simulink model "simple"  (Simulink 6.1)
settings: Solver=ode45  StartTime=0.0  StopTime=25.0  RelTol=1e-3
undefined symbols (not defined in the file or in its folder): Bit, Location, Lower, netlist, Width
libraries: xbsIndex_r3 x16, adlibrary2 x1

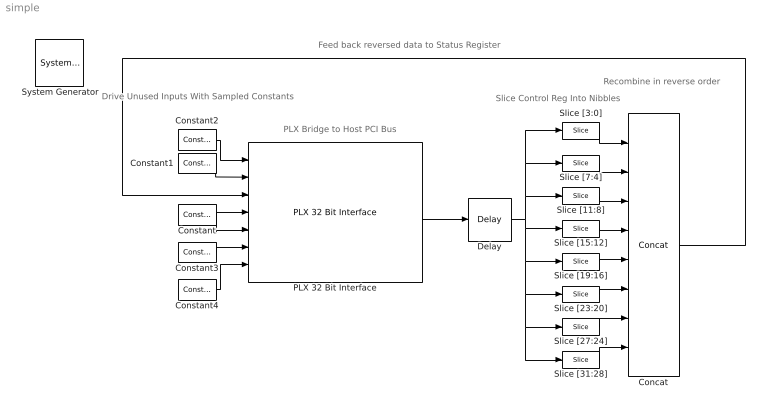
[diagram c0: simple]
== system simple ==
  note: Drive Unused Inputs With Sampled Constants
  note: PLX Bridge to Host PCI Bus
  note: Slice Control Reg Into Nibbles
  note: Recombine in reverse order
  note: Feed back reversed data to Status Register
  " System Generator" : xbsIndex_r3/ System Generator  Tag=genX  xilinxfamily=Virtex4  part=xc4vsx55  speed=-10  package=ff1148  synthesis_tool=XST  directory=./netlist  testbench=off  simulink_period=1  sysclk_period=10  incr_netlist=off  trim_vbits=Everywhere in SubSystem  dbl_ovrd=According to Block Masks  core_generation=According to Block Masks  run_coregen=off  deprecated_control=off  eval_field=0
  Concat : xbsIndex_r3/Concat  num_inputs=8  explicit_period=off  period=1  dbl_ovrd=off
  Constant : xbsIndex_r3/Constant  const=0  equ=P=C  arith_type=Boolean  n_bits=1  bin_pt=0  opselect=C  inp2=PCIN>>17  opr=+  inp1=P  carry=CIN  iostate=0  explicit_period=on  period=1  dbl_ovrd=off
  Constant1 : xbsIndex_r3/Constant  const=1  equ=P=C  arith_type=Boolean  n_bits=1  bin_pt=0  opselect=C  inp2=PCIN>>17  opr=+  inp1=P  carry=CIN  iostate=0  explicit_period=on  period=1  dbl_ovrd=off
  Constant2 : xbsIndex_r3/Constant  const=0  equ=P=C  arith_type=Unsigned  n_bits=32  bin_pt=0  opselect=C  inp2=PCIN>>17  opr=+  inp1=P  carry=CIN  iostate=0  explicit_period=on  period=1  dbl_ovrd=off
  Constant3 : xbsIndex_r3/Constant  const=0  equ=P=C  arith_type=Unsigned  n_bits=32  bin_pt=0  opselect=C  inp2=PCIN>>17  opr=+  inp1=P  carry=CIN  iostate=0  explicit_period=on  period=1  dbl_ovrd=off
  Constant4 : xbsIndex_r3/Constant  const=0  equ=P=C  arith_type=Unsigned  n_bits=34  bin_pt=0  opselect=C  inp2=PCIN>>17  opr=+  inp1=P  carry=CIN  iostate=0  explicit_period=on  period=1  dbl_ovrd=off
  Delay : xbsIndex_r3/Delay  latency=1  reg_retiming=off  explicit_period=on  period=1  en=off  accept_only_valid=off  init_zero=on  dbl_ovrd=off  show_param=off
  PLX 32 Bit Interface : adlibrary2/ADM-XRC-II/PLX 32 Bit Interface  program='slave_write 0x40000 0xabcd1234;slave_read 0x40040'  clock_ratio=1.5
  Slice [11:8] : xbsIndex_r3/Slice  mode=Lower Bit Location + Width  nbits=4  bit1=0  base1=MSB of Input  bit0=8  base0=LSB of Input  boolean_output=off  explicit_period=off  period=1  dbl_ovrd=off
  Slice [15:12] : xbsIndex_r3/Slice  mode=Lower Bit Location + Width  nbits=4  bit1=0  base1=MSB of Input  bit0=12  base0=LSB of Input  boolean_output=off  explicit_period=off  period=1  dbl_ovrd=off
  Slice [19:16] : xbsIndex_r3/Slice  mode=Lower Bit Location + Width  nbits=4  bit1=0  base1=MSB of Input  bit0=16  base0=LSB of Input  boolean_output=off  explicit_period=off  period=1  dbl_ovrd=off
  Slice [23:20] : xbsIndex_r3/Slice  mode=Lower Bit Location + Width  nbits=4  bit1=0  base1=MSB of Input  bit0=20  base0=LSB of Input  boolean_output=off  explicit_period=off  period=1  dbl_ovrd=off
  Slice [27:24] : xbsIndex_r3/Slice  mode=Lower Bit Location + Width  nbits=4  bit1=0  base1=MSB of Input  bit0=24  base0=LSB of Input  boolean_output=off  explicit_period=off  period=1  dbl_ovrd=off
  Slice [31:28] : xbsIndex_r3/Slice  mode=Lower Bit Location + Width  nbits=4  bit1=0  base1=MSB of Input  bit0=28  base0=LSB of Input  boolean_output=off  explicit_period=off  period=1  dbl_ovrd=off
  Slice [3:0] : xbsIndex_r3/Slice  mode=Lower Bit Location + Width  nbits=4  bit1=0  base1=MSB of Input  bit0=0  base0=LSB of Input  boolean_output=off  explicit_period=off  period=1  dbl_ovrd=off
  Slice [7:4] : xbsIndex_r3/Slice  mode=Lower Bit Location + Width  nbits=4  bit1=0  base1=MSB of Input  bit0=4  base0=LSB of Input  boolean_output=off  explicit_period=off  period=1  dbl_ovrd=off
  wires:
  Constant/1 -> PLX 32 Bit Interface/4, PLX 32 Bit Interface/5
  Constant1/1 -> PLX 32 Bit Interface/2
  Constant2/1 -> PLX 32 Bit Interface/1
  Constant3/1 -> PLX 32 Bit Interface/6
  Constant4/1 -> PLX 32 Bit Interface/7
  PLX 32 Bit Interface/6 -> Delay/1
  Delay/1 -> Slice [31:28]/1, Slice [27:24]/1, Slice [23:20]/1, Slice [19:16]/1, Slice [15:12]/1, Slice [11:8]/1, Slice [3:0]/1, Slice [7:4]/1
  Slice [3:0]/1 -> Concat/1
  Slice [7:4]/1 -> Concat/2
  Slice [11:8]/1 -> Concat/3
  Slice [15:12]/1 -> Concat/4
  Slice [19:16]/1 -> Concat/5
  Slice [23:20]/1 -> Concat/6
  Slice [27:24]/1 -> Concat/7
  Slice [31:28]/1 -> Concat/8
  Concat/1 -> PLX 32 Bit Interface/3
